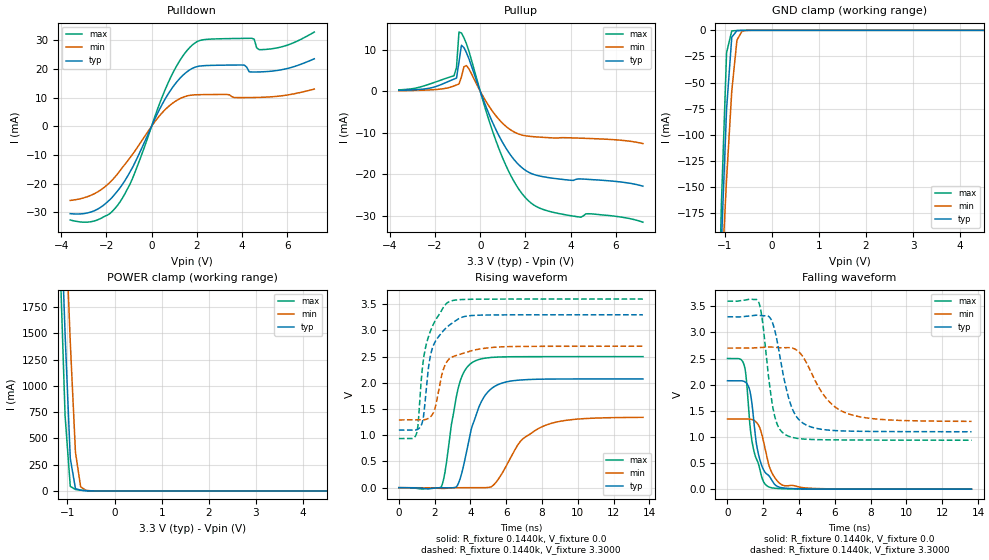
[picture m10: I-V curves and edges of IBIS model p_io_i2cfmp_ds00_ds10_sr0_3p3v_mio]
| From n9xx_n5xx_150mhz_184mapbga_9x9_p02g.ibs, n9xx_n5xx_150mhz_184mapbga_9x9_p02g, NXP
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[Model] p_io_i2cfmp_ds00_ds10_sr0_3p3v_mio
|   Model p_io_i2cfmp_ds00_ds10_sr0_3p3v_mio
| This model was characterised for following simulation conditions:
| External (pad) voltage:
|   - Typ: 3.3V,   - Min: 2.7V,   - Max: 3.6V
| Library cells for typ/min/max conditions are connected as defined below:
|  pad - External Pad
|  ipp_do_lv - Core Input
|  ipp_obe_lv - Output Buffer Enable
|  IOGC - NC
|  REFH3V3 - REFH3V3
|  REFL3V3 - REFL3V3
|  ZI - NC
|  abut_ncal_vddio[1] - vddio
|  abut_ncal_vddio[2] - vddio
|  abut_ncal_vddio[3] - vssio
|  abut_ncal_vddio[4] - vddio
|  abut_ncal_vddio[5] - vddio
|  abut_ncal_vddio[6] - vssio
|  abut_pcal_vddio[1] - vssio
|  abut_pcal_vddio[2] - vssio
|  abut_pcal_vddio[3] - vddio
|  abut_pcal_vddio[4] - vssio
|  abut_pcal_vddio[5] - vssio
|  abut_pcal_vddio[6] - vddio
|  ipp_do_1p8v - ipp_do_1p8v
|  ipp_dse_lv[0] - 0
|  ipp_dse_lv[1] - 0
|  ipp_eftd_lv - NC
|  ipp_ina_mux_vddio - NC
|  ipp_ina_mux_vddio[0] - NC
|  ipp_ina_mux_vddio[1] - NC
|  ipp_ina_r0_vddio - NC
|  ipp_ina_r0a_vddio - NC
|  ipp_ina_r0b_vddio - NC
|  ipp_ina_r0c_vddio - NC
|  ipp_ina_r0d_vddio - NC
|  ipp_ina_r0e_vddio - NC
|  ipp_ina_r0f_vddio - NC
|  ipp_ina_r300_vddio - NC
|  ipp_ina_r300a_vddio - NC
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Model_type I/O
Polarity   Non-Inverting
Enable   Active-High
Vinl =   0.9900V
Vinh =   2.3100V
Vmeas =  1.6500V
Cref =   30.0000pF
Rref =   1.0000M
Vref =   3.3000V
C_comp   1.7403pF   1.7015pF   1.7922pF
|C_comp_pullup   0.6949pF   0.7584pF   0.6579pF
|C_comp_pulldown   0.9320pF   0.9172pF   0.9310pF
[Model Spec]
| variable   typ   min   max
Vinh   2.3100V   1.8900V   2.5200V
Vinl   0.9900V   0.8100V   1.0800V
[Temperature Range]   25.0000   0.1250k   -40.0000
[Voltage Range]   3.3000V   2.7000V   3.6000V
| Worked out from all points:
|   slope of the pulldown table from 0 to 0.495 V, typ, clamps not added: 61.7 ohm
|   slope of the pullup table from 0 to 0.495 V, typ, clamps not added: 72.2 ohm
|   GND clamp passes 1 mA (typ) near -0.75 V on its own axis
|   POWER clamp passes 1 mA (typ) near -0.52 V on its own axis
|   rising waveform, R_fixture 0.1440k, V_fixture 0.0: 20-80 % time 1.03ns typ, 1.78ns min, 728ps max; typ from 0 V to 2.08 V
|   rising waveform, R_fixture 0.1440k, V_fixture 3.3000: 20-80 % time 732ps typ, 649ps min, 726ps max; typ from 1.1 V to 3.3 V
|   falling waveform, R_fixture 0.1440k, V_fixture 0.0: 20-80 % time 596ps typ, 652ps min, 636ps max; typ from 2.08 V to 0 V
|   falling waveform, R_fixture 0.1440k, V_fixture 3.3000: 20-80 % time 861ps typ, 1.58ns min, 580ps max; typ from 3.3 V to 1.1 V
[Pulldown]
|Voltage   I(typ)   I(min)   I(max)
-3.6V     -30.44mA   -25.83mA   -32.65mA
-2.39V    -28.88mA   -22.87mA   -32.61mA
-1.4V     -21.46mA   -15.51mA   -26.39mA
-850mV    -14.46mA   -9.856mA   -18.31mA
800mV     12.05mA    7.226mA    16.28mA
1.35V     17.48mA    9.968mA    24.09mA
1.9V      20.5mA     10.93mA    28.91mA
4.1V      21.31mA    9.981mA    30.6mA
4.43V     18.9mA     10mA       30.65mA
4.65V     18.9mA     10.03mA    27.3mA
5.09V     19.05mA    10.15mA    26.78mA
7.2V      23.49mA    12.94mA    32.8mA
[Pullup]
|Voltage   I(typ)   I(min)   I(max)
-3.6V     205.5uA    122.8uA    318.7uA
-1.16V    2.91mA     1.263mA    3.707mA
-1.05V    3.138mA    1.494mA    5.669mA
-940mV    6.993mA    1.733mA    14.21mA
-830mV    11.04mA    3.449mA    14mA
-720mV    10.47mA    5.872mA    12.85mA
-610mV    9.27mA     6.173mA    11.42mA
820mV     -10.6mA    -6.722mA   -13.7mA
1.48V     -16.32mA   -9.741mA   -21.54mA
2.03V     -19.11mA   -10.73mA   -25.77mA
3.46V     -21.08mA   -11.23mA   -29.38mA
7.2V      -22.83mA   -12.59mA   -31.48mA
[GND_clamp]
|Voltage   I(typ)   I(min)   I(max)
-3.6V     -4.377A    -3.283A    -5.855A
-1.18V    -351.7mA   -346.5mA   -367.9mA
-1.07V    -204.2mA   -241.2mA   -166.2mA
-960mV    -75.42mA   -142.6mA   -21.4mA
-850mV    -6.575mA   -58.21mA   -529.8uA
-740mV    -281.6uA   -9.383mA   -183.8uA
-630mV    -73.66uA   -605.1uA   -74.76uA
-410mV    -3.148uA   -9.219uA   -1.868uA
7.2V      0A         0A         0A
[POWER_clamp]
|Voltage   I(typ)   I(min)   I(max)
-3.6V     34.56A     31.8A      37.41A
-1.16V    2.902A     3.904A     2.233A
-1.05V    1.495A     2.658A     715.5mA
-940mV    310.6mA    1.419A     44.07mA
-830mV    22.38mA    368.3mA    13.28mA
-720mV    6.713mA    39.84mA    7.005mA
-610mV    2.702mA    5.591mA    2.612mA
7.2V      0A         0A         0A
[Ramp]
| variable   typ   min   max
dV/dt_r  1.2454/1.0255n   0.8053/1.7792n   1.5009/0.7276n
dV/dt_f  1.3205/0.8610n   0.8413/1.5813n   1.5977/0.5797n
R_load = 0.1440k
[Rising Waveform]
R_fixture= 0.1440k
V_fixture= 0.0
V_fixture_min= 0.0
V_fixture_max= 0.0
|time   V(typ)   V(min)   V(max)
0s        5.868nV    472.7nV    20.52nV
2.377ns   -1.721mV   -16.04mV   22.87mV
2.573ns   -2.094mV   -12.38mV   285.2mV
3.366ns   113.7mV    -802.2uV   1.964V
4.228ns   1.294V     -2.108mV   2.414V
4.773ns   1.739V     -921.4uV   2.47V
5.429ns   1.949V     101.6mV    2.491V
6.811ns   2.056V     891.2mV    2.501V
8.152ns   2.072V     1.185V     2.501V
13.64ns   2.076V     1.342V     2.502V
[Rising Waveform]
R_fixture= 0.1440k
V_fixture= 3.3000
V_fixture_min= 2.7000
V_fixture_max= 3.6000
|time   V(typ)   V(min)   V(max)
0s        1.098V     1.293V     936.9mV
969.7ps   1.102V     1.293V     1.014V
1.081ns   1.119V     1.294V     1.239V
1.32ns    1.26V      1.294V     2.299V
1.52ns    1.843V     1.303V     2.718V
1.884ns   2.674V     1.403V     3.086V
2.454ns   2.982V     2.223V     3.423V
2.757ns   3.085V     2.438V     3.54V
5.401ns   3.297V     2.682V     3.599V
13.64ns   3.3V       2.7V       3.6V
[Falling Waveform]
R_fixture= 0.1440k
V_fixture= 0.0
V_fixture_min= 0.0
V_fixture_max= 0.0
|time   V(typ)   V(min)   V(max)
0s        2.076V     1.344V     2.502V
920.4ps   2.065V     1.343V     2.387V
1.051ns   2.033V     1.343V     2.118V
1.23ns    1.91V      1.342V     1.322V
1.426ns   1.46V      1.325V     810.9mV
1.59ns    935.2mV    1.288V     600.3mV
1.76ns    627.9mV    1.209V     449.9mV
2.283ns   268.5mV    497.1mV    47.53mV
3.233ns   19.5mV     63.81mV    7.384mV
13.64ns   7.221uV    77.89uV    956.4nV
[Falling Waveform]
R_fixture= 0.1440k
V_fixture= 3.3000
V_fixture_min= 2.7000
V_fixture_max= 3.6000
|time   V(typ)   V(min)   V(max)
0s        3.3V       2.7V       3.6V
1.736ns   3.33V      2.71V      3.587V
1.943ns   3.319V     2.714V     3.251V
2.564ns   3.14V      2.718V     1.513V
3.247ns   1.98V      2.709V     1.042V
3.657ns   1.511V     2.697V     987.9mV
4.159ns   1.279V     2.563V     961.8mV
5.44ns    1.137V     1.773V     945.3mV
6.554ns   1.113V     1.468V     941.7mV
13.64ns   1.099V     1.298V     937.1mV
